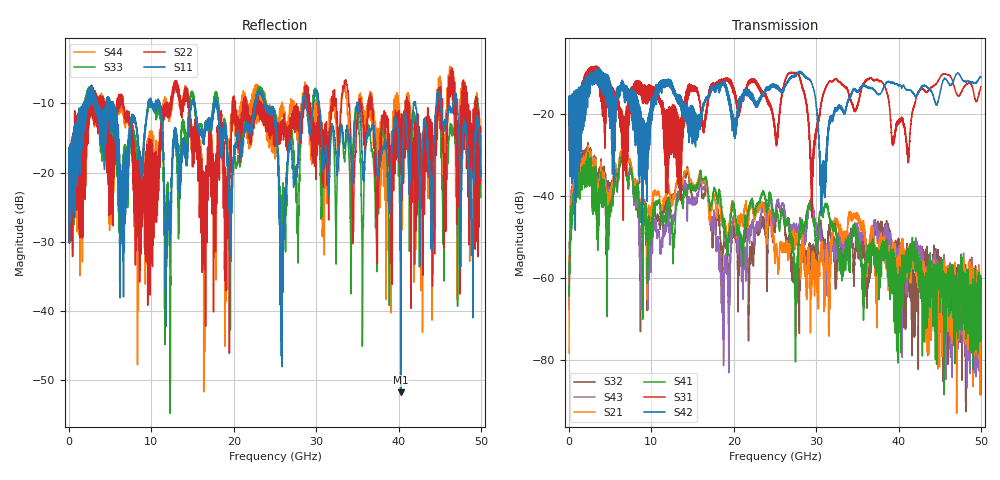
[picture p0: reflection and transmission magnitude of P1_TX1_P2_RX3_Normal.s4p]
!Keysight Technologies,N5225B,MY57041031,A.13.20.10
!Date: Friday, May 31, 2019 11:31:35
!Correction: S11(Full 4 Port(1,2,3,4))
!S12(Full 4 Port(1,2,3,4))
!S13(Full 4 Port(1,2,3,4))
!S14(Full 4 Port(1,2,3,4))
!S21(Full 4 Port(1,2,3,4))
!S22(Full 4 Port(1,2,3,4))
!S23(Full 4 Port(1,2,3,4))
!S24(Full 4 Port(1,2,3,4))
!S31(Full 4 Port(1,2,3,4))
!S32(Full 4 Port(1,2,3,4))
!S33(Full 4 Port(1,2,3,4))
!S34(Full 4 Port(1,2,3,4))
!S41(Full 4 Port(1,2,3,4))
!S42(Full 4 Port(1,2,3,4))
!S43(Full 4 Port(1,2,3,4))
!S44(Full 4 Port(1,2,3,4))
!S4P File: Measurements: <S11,S12,S13,S14>,
!<S21,S22,S23,S24>,
!<S31,S32,S33,S34>,
!<S41,S42,S43,S44>:
# Hz S  dB  R 50.0
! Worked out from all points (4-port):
!   5000 points, 10 MHz to 50 GHz, reference 50 ohm
!   strongest paths, dB at 10 MHz, 12.51 GHz, 25.01 GHz, 37.51 GHz, 50 GHz:
!     S42: -19.4, -14.3, -13.2, -15.4, -11.2
!     S31: -19.5, -29.2, -24.6, -11.8, -13.5
!     S41: -62.0, -47.6, -45.5, -54.3, -60.1
!     S21: -78.3, -42.0, -56.5, -59.0, -62.9
!     S43: -66.6, -47.6, -44.7, -49.5, -68.7
!     S32: -67.7, -40.9, -47.4, -47.7, -60.6
!   lowest |S11| = -51.7 dB at 40.27 GHz (marker M1), VSWR 1.01, Z = 49.8 + j0.171 ohm
!   |S11| at or under -10 dB: 18.01 GHz to 22.61 GHz (4.596 GHz wide, 22.6 % of centre); 30.38 GHz to 34.94 GHz (4.562 GHz wide, 14 % of centre); 34.98 GHz to 41.81 GHz (6.839 GHz wide, 17.8 % of centre)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
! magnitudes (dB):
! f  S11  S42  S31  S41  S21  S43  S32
! 10 MHz  -19.9  -19.4  -19.5  -62.0  -78.3  -66.6  -67.7
! 960 MHz  -17.1  -19.7  -19.3  -35.5  -33.3  -33.3  -31.0
! 6.38 GHz  -23.7  -13.1  -22.0  -30.7  -29.5  -30.9  -30.2
! 28.19 GHz  -11.9  -9.9  -12.6  -46.6  -54.3  -47.7  -51.9
! 30.79 GHz  -18.1  -31.7  -16.1  -45.3  -54.7  -51.6  -50.1
! 40.27 GHz  -51.7  -13.2  -21.4  -78.2  -58.3  -63.6  -57.1
! 50 GHz  -19.6  -11.2  -13.5  -60.1  -62.9  -68.7  -60.6
